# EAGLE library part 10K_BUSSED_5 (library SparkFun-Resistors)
5 x 10kΩ resistor network A resistor is a passive two-terminal electrical component that implements electrical resistance as a circuit element. Resistors act to reduce current flow, and, at the same time, act to lower voltage levels within circuits. - Wikipedia This is a bussed or ladder network.
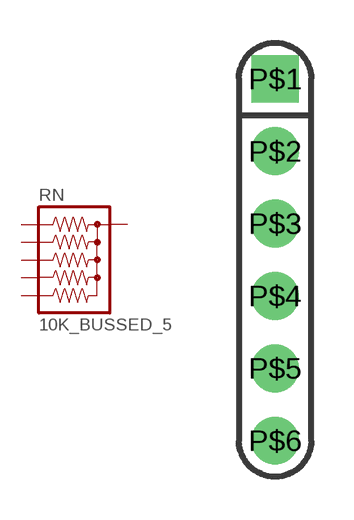
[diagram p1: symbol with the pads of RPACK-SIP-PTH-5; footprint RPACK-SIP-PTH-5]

Designator prefix RN

## 10K_BUSSED_5 (SF_SKU: COM-10856; VALUE: 10k)  [RPACK-SIP-PTH-5]
P$1  1  pas
P$2  2  pas
P$3  3  pas
P$4  4  pas
P$5  5  pas
P$6  6  pas

## Footprint RPACK-SIP-PTH-5 (pad centres in mm)
Based on this datasheet.
drill 0.8 pad 1.676 square: P$1 0,0
drill 0.8 pad 1.676: P$2 0,-2.54; P$3 0,-5.08; P$4 0,-7.62; P$5 0,-10.16; P$6 0,-12.7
